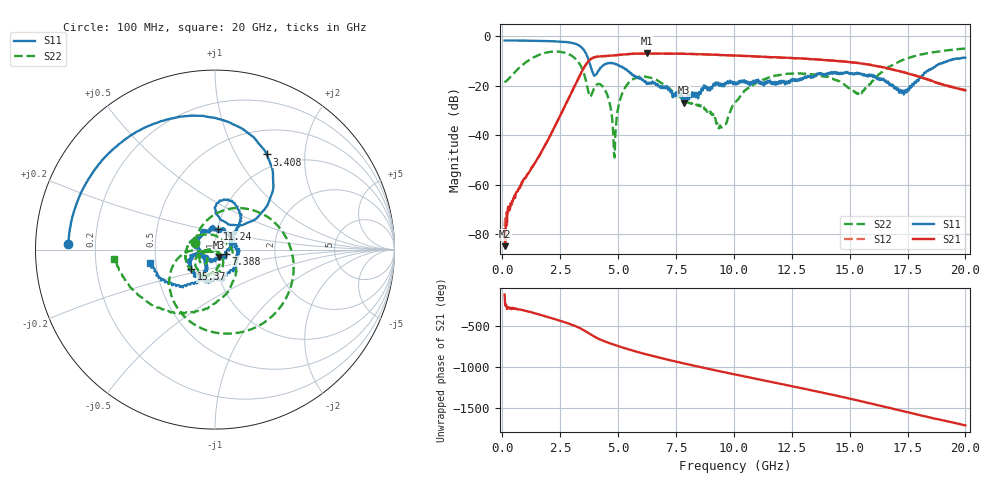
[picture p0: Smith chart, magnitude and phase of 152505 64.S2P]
!  2-Port S-parameters saved by WinCal
! VAR MeasName=S-Parameters (CALIBRATED_DATA) read from VNA (N5230C)
! VAR MeasDate=4/10/2015 9:35:20 AM
! VAR NAME=152505 64
! VAR FILENAME=152505 64.S2P
! VAR DATE=4/10/2015 9:35:20 AM
! VAR PHYS_PORTS=1,2
# Hz S DB R 50
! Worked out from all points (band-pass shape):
!   801 points, 100 MHz to 20 GHz, reference 50 ohm
!   highest |S21| = -6.99 dB at 6.244 GHz (marker M1); lowest = -84.7 dB at 124.9 MHz (marker M2)
!   |S21| within 3 dB of the highest: 3.734 GHz to 14.4 GHz (10.66 GHz wide, 118 % of centre)
!   lowest |S11| = -26.9 dB at 7.861 GHz (marker M3), VSWR 1.10, Z = 51.9 - j4.24 ohm
!   |S11| at or under -10 dB: 3.742 GHz to 19.24 GHz (15.5 GHz wide, 135 % of centre)
!   |S22| runs from -48.9 to -5.0 dB; largest |S21 - S12| = 0.0057
!   S11 on the Smith chart (normalised r, x): 100 MHz: 0.10, +0.02; 3.408 GHz: 0.81, +1.35; 7.388 GHz: 1.13, -0.05; 11.24 GHz: 1.00, +0.23; 15.37 GHz: 0.75, -0.17; 20 GHz: 0.47, -0.08
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1e8  -1.75 177.6  -77.87 -125.8  -76.69 66.1  -18.64 161.5
1.24875e8  -1.75 177.0  -84.71 100.6  -73.50 77.6  -18.47 156.8
1.816375e9  -1.98 134.5  -44.49 -25.4  -44.51 -25.4  -6.85 -15.6
2.612375e9  -2.28 108.0  -29.91 -92.8  -29.99 -93.1  -6.51 -82.2
3.408375e9  -4.38 61.4  -14.73 179.9  -14.74 -179.9  -12.35 -161.0
3.43325e9  -4.62 59.6  -14.29 176.4  -14.29 176.5  -12.83 -163.7
3.7815e9  -11.11 36.8  -9.56 118.4  -9.58 118.4  -24.36 -151.8
4.453125e9  -11.21 84.6  -8.03 24.6  -8.07 24.4  -22.04 -164.2
4.851125e9  -11.06 66.7  -7.75 -15.0  -7.74 -15.2  -48.89 -52.4
5.298875e9  -13.31 49.8  -7.34 -55.1  -7.36 -54.9  -20.88 -60.5
6.244125e9  -19.34 38.7  -6.99 -130.8  -7.04 -130.9  -16.56 -126.8
6.741625e9  -20.28 31.9  -7.03 -165.9  -7.04 -166.0  -18.14 -152.8
7.388375e9  -23.68 -20.2  -7.06 150.6  -7.06 150.6  -22.61 -168.3
7.861e9  -26.86 -63.9  -7.15 120.1  -7.12 120.4  -25.93 -165.2
9.428125e9  -19.13 167.4  -7.61 24.5  -7.63 24.4  -36.53 -117.6
1.005e10  -18.68 141.5  -7.83 -11.7  -7.86 -12.0  -26.71 -60.5
1.1244e10  -18.71 83.1  -8.30 -80.4  -8.32 -80.4  -17.59 -96.7
1.338325e10  -16.26 -57.4  -9.31 155.0  -9.25 155.5  -15.38 -167.9
1.537325e10  -15.26 -140.9  -10.88 32.6  -10.84 32.5  -23.08 56.2
1.669162e10  -19.04 -162.5  -13.09 -54.5  -13.14 -55.2  -12.43 -70.8
1.743788e10  -22.59 -130.8  -14.81 -104.0  -14.92 -103.6  -9.20 -103.5
2e10  -8.67 -168.2  -21.86 91.7  -21.87 92.0  -4.99 -174.6
